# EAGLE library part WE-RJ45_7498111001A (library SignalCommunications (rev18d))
Order Code 7498111001A Design SMD xBase-T 10/100/1000 Base-T Ports 1x1 Application Standard Tab Position UP LED (Left-Right) NONE EMI Fingers Yes Details see: http://katalog.we-online.de/en/pbs/WE-LAN_RJ45 Created by Yingchun Shan 2016-08-23 2016 (C) Würth Elektronik
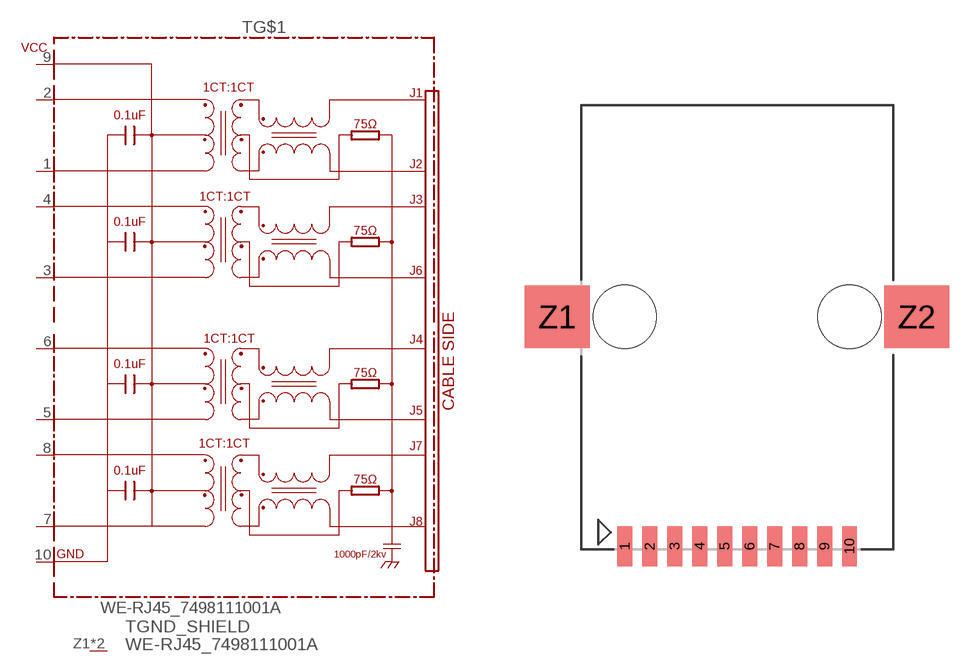
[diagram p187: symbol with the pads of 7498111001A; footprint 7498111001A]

Designator prefix T; gates G$1=7498111001A GND_SHIELD=GNDPIN

## WE-RJ45_7498111001A  [7498111001A]
1  G$1:1
2  G$1:2
3  G$1:3
4  G$1:4
5  G$1:5
6  G$1:6
7  G$1:7
8  G$1:8
9  G$1:VCC
10  G$1:GND
Z1  GND_SHIELD:GND  pwr
Z2  GND_SHIELD:GND  pwr

## Footprint 7498111001A (pad centres in mm)
smd 0.76 x 2.03: 1 -5.715,-11.68; 2 -4.445,-11.68; 3 -3.175,-11.68; 4 -1.905,-11.68; 5 -0.635,-11.68; 6 0.635,-11.68; 7 1.905,-11.68; 8 3.175,-11.68; 9 4.445,-11.68; 10 5.715,-11.68
smd 3.3 x 3.18: Z1 -9.145,0; Z2 9.145,0
hole 3.22 at -5.715,0
hole 3.22 at 5.715,0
